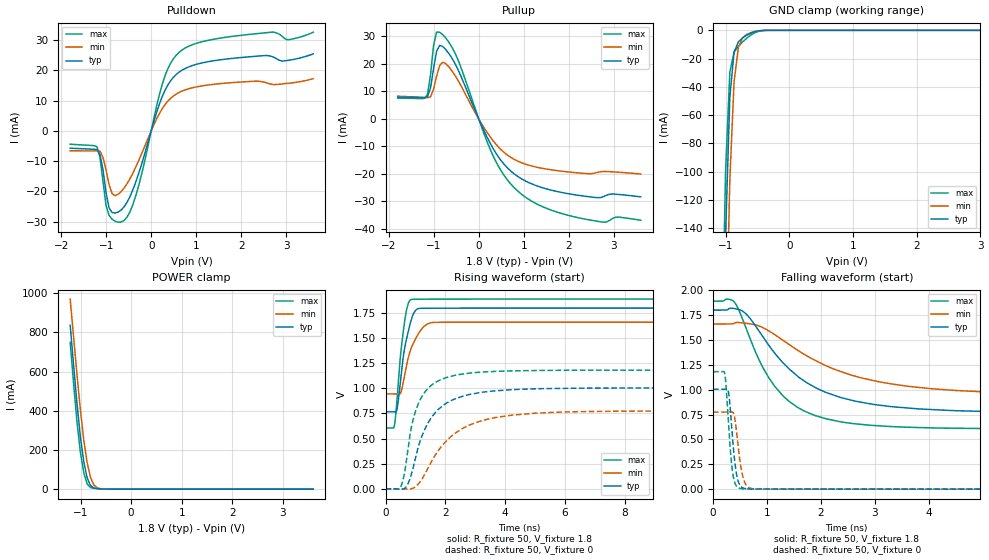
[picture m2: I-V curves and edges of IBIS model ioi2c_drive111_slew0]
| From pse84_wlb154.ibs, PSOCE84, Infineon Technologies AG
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[Model] ioi2c_drive111_slew0
Model_type I/O
Enable   Active-High
Vinl  =  0.54
Vinh  =  1.26
Vmeas =  0.9
Cref  =  15e-12
| Capacitance   typ   min   max
C_comp   8.55364e-13 8.30808e-13 8.84570e-13
| Variables   typ   min   max
[GND Clamp Reference]   0   0   0
[POWER Clamp Reference]   1.8   1.66   1.89
[Pulldown Reference]   0   0   0
[Pullup Reference]   1.8   1.66   1.89
[Temperature Range]   25   125   -40
[Voltage Range]   1.8   1.66   1.89
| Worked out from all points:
|   slope of the pulldown table from 0 to 0.27 V, typ, clamps not added: 22.3 ohm
|   slope of the pullup table from 0 to 0.27 V, typ, clamps not added: 29.1 ohm
|   GND clamp passes 1 mA (typ) near -0.55 V on its own axis
|   POWER clamp passes 1 mA (typ) near -0.55 V on its own axis
|   falling waveform, R_fixture 50, V_fixture 1.8: 20-80 % time 1.24ns typ, 1.76ns min, 863ps max; typ from 1.8 V to 0.767 V
|   falling waveform, R_fixture 50, V_fixture 0: 20-80 % time 101ps typ, 115ps min, 93.8ps max; typ from 1 V to 0 V
|   rising waveform, R_fixture 50, V_fixture 1.8: 20-80 % time 316ps typ, 436ps min, 245ps max; typ from 0.767 V to 1.8 V
|   rising waveform, R_fixture 50, V_fixture 0: 20-80 % time 902ps typ, 1.37ns min, 594ps max; typ from 0 V to 1 V
[GND Clamp]
| Voltage   I(typ)   I(min)   I(max)
-1.204V   -750.5mA   -844.3mA   -692.2mA
-1.07V    -311.8mA   -416.8mA   -250.3mA
-1.003V   -144.6mA   -236.7mA   -99.35mA
-936.6mV  -47.15mA   -105.3mA   -29.57mA
-869.7mV  -15.32mA   -36.11mA   -15.4mA
-802.8mV  -8.178mA   -12.13mA   -11.32mA
-735.9mV  -5.345mA   -5.294mA   -8.218mA
-669mV    -3.361mA   -2.852mA   -5.471mA
-535.2mV  -838.5uA   -772.4uA   -1.486mA
-401.4mV  -47.36uA   -84.85uA   -76.78uA
3.6V      0A         0A         0A
[POWER Clamp]
| Voltage   I(typ)   I(min)   I(max)
-1.204V   837.3mA    970.7mA    749.2mA
-1.137V   634.9mA    778.2mA    540.5mA
-1.07V    440.1mA    587.4mA    346.5mA
-1.003V   270mA      407mA      190.9mA
-936.6mV  141.8mA    252.7mA    85.92mA
-869.7mV  58.74mA    136.5mA    26.66mA
-802.8mV  18.35mA    60.36mA    8.197mA
-735.9mV  5.885mA    21mA       4.755mA
-669mV    2.866mA    6.628mA    3.138mA
-334.5mV  12.31uA    45.7uA     5.857uA
3.6V      0A         0A         0A
[Pulldown]
| Voltage   I(typ)   I(min)   I(max)
-1.8V     -5.733mA   -6.58mA    -4.413mA
-1.204V   -6.136mA   -6.633mA   -5.256mA
-1.07V    -12.91mA   -8.837mA   -16.72mA
-1.003V   -20.35mA   -12.88mA   -24.6mA
-936.6mV  -25.37mA   -17.69mA   -27.84mA
-802.8mV  -27.11mA   -21.39mA   -29.8mA
-669mV    -26.13mA   -20.06mA   -30.09mA
-334.5mV  -16.53mA   -11.66mA   -21.01mA
310.3mV   13.46mA    8.709mA    18.26mA
620.7mV   19.37mA    12.66mA    25.9mA
1.614V    23.57mA    15.67mA    30.76mA
3.6V      25.4mA     17.19mA    32.53mA
[Pullup]
| Voltage   I(typ)   I(min)   I(max)
-1.8V     7.983mA    8.276mA    7.55mA
-1.137V   8.081mA    7.705mA    8.92mA
-1.07V    11.29mA    8.026mA    16.09mA
-1.003V   18.26mA    10.85mA    26.69mA
-936.6mV  24.58mA    15.49mA    31.57mA
-869.7mV  26.74mA    19.33mA    31.53mA
-735.9mV  25.28mA    20.15mA    29.47mA
-468.3mV  18.22mA    14.26mA    21.82mA
372.4mV   -12.19mA   -9.009mA   -15.2mA
869mV     -20.94mA   -15.36mA   -26.26mA
2.126V    -27.56mA   -19.51mA   -35.61mA
3.6V      -28.34mA   -20.03mA   -36.86mA
[Ramp]
dV/dt_r   0.6024/0.901598n  0.4646/1.36683n  0.708544/0.59385n
dV/dt_f   0.619731/1.24185n  0.429004/1.76088n  0.77075/0.862698n
R_load = 50
[Falling Waveform]
R_fixture = 50
V_fixture = 1.8
V_fixture_min = 1.66
V_fixture_max = 1.89
| Time   V(typ)   V(min)   V(max)
0s        1.8V       1.66V      1.89V
387.6ps   1.816V     1.668V     1.885V
623.2ps   1.756V     1.667V     1.601V
842.7ps   1.597V     1.642V     1.312V
1.146ns   1.367V     1.553V     1.032V
1.884ns   1.026V     1.298V     741.6mV
2.654ns   883mV      1.133V     656.3mV
3.623ns   815.5mV    1.034V     622.4mV
6.43ns    771.4mV    957.2mV    605.3mV
800ns     767.1mV    945mV      605.4mV
[Falling Waveform]
R_fixture = 50
V_fixture = 0
V_fixture_min = 0
V_fixture_max = 0
| Time   V(typ)   V(min)   V(max)
0s        1.004V     774.3mV    1.181V
217.4ps   1.004V     774.3mV    1.159V
242.7ps   1.004V     774.3mV    1.03V
294.6ps   946.3mV    774.2mV    577.9mV
347.7ps   601mV      775.8mV    232mV
408.1ps   253mV      695mV      57.64mV
477.7ps   61.11mV    367.9mV    11.42mV
583.5ps   7.364mV    72.82mV    2.306mV
957.6ps   1.27mV     1.56mV     793.6uV
800ns     6.177nV    431nV      2.268nV
[Rising Waveform]
R_fixture = 50
V_fixture = 1.8
V_fixture_min = 1.66
V_fixture_max = 1.89
| Time   V(typ)   V(min)   V(max)
0s        767.1mV    945mV      605.4mV
299.4ps   767.3mV    945mV      635.5mV
391.2ps   804.6mV    945.1mV    916.9mV
517.1ps   1.123V     962.9mV    1.376V
624.2ps   1.376V     1.109V     1.637V
745.7ps   1.549V     1.287V     1.834V
890.4ps   1.712V     1.425V     1.887V
998.2ps   1.775V     1.49V      1.888V
1.369ns   1.798V     1.636V     1.889V
800ns     1.8V       1.66V      1.89V
[Rising Waveform]
R_fixture = 50
V_fixture = 0
V_fixture_min = 0
V_fixture_max = 0
| Time   V(typ)   V(min)   V(max)
0s        6.178nV    430.8nV    2.27nV
519.7ps   -3.541mV   -1.525mV   26.9mV
720.1ps   33.09mV    -2.819mV   326mV
922.3ps   208.9mV    6.206mV    689.3mV
1.31ns    589.8mV    142.8mV    962.1mV
1.634ns   748.6mV    321.5mV    1.053V
2.083ns   861mV      490.9mV    1.112V
3.188ns   959.6mV    674.4mV    1.162V
7.769ns   1.004V     772.6mV    1.181V
50ns      1.004V     774.3mV    1.181V
